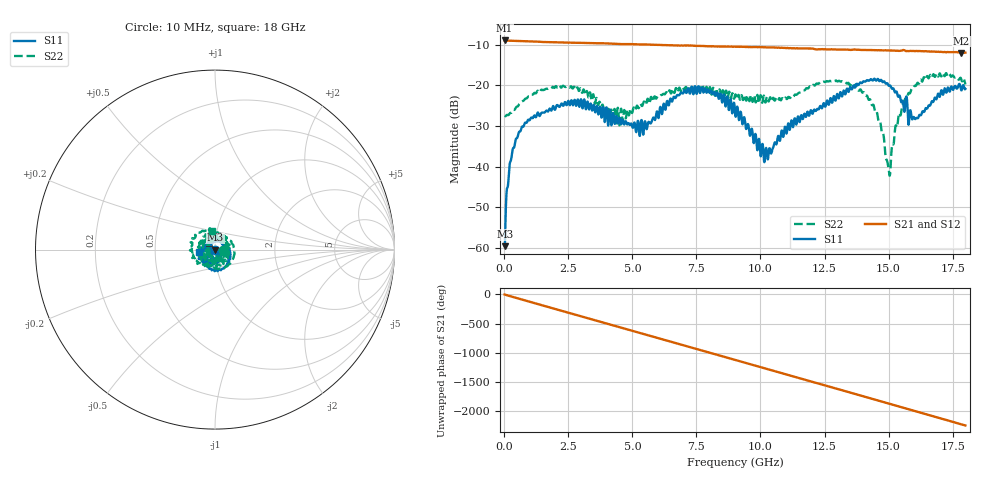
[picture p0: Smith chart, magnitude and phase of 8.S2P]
!Agilent Technologies,E5071C,MY46316741,A.11.02
!Date: Fri May 06 15:19:51 2022
!Data & Calibration Information:
!Freq	S11:SOLT2(ON)	S21:SOLT2(ON)	S12:SOLT2(ON)	S22:SOLT2(ON)
!PortZ  Port1:50+j0  Port2:50+j0
!Above PortZ is port z conversion or system Z0 setting when saving the data.
!When reading, reference impedance value at option line is always used.
# Hz S dB R 50
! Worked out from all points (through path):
!   1800 points, 10 MHz to 18 GHz, reference 50 ohm
!   highest |S21| = -8.93 dB at 10 MHz (marker M1); lowest = -12.0 dB at 17.84 GHz (marker M2)
!   group delay of S21, straight-line fit = 346 ps
!   lowest |S11| = -59.6 dB at 20 MHz (marker M3), VSWR 1.00, Z = 50.1 - j0.0653 ohm
!   |S11| at or under -10 dB: start of sweep to end of sweep
!   |S22| runs from -42.2 to -17.0 dB; largest |S21 - S12| = 0.021
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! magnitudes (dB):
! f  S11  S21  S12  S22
! 10 MHz  -59.1  -8.9  -8.9  -27.5
! 20 MHz  -59.6  -8.9  -8.9  -27.5
! 150 MHz  -44.1  -9.0  -9.0  -27.3
! 260 MHz  -38.3  -9.0  -9.0  -26.7
! 640 MHz  -31.1  -9.1  -9.1  -24.4
! 3.01 GHz  -23.8  -9.5  -9.5  -21.4
! 4.43 GHz  -29.4  -9.8  -9.8  -25.5
! 5.35 GHz  -28.5  -9.9  -9.9  -24.9
! 6.01 GHz  -27.9  -10.0  -10.0  -22.6
! 7.51 GHz  -22.1  -10.3  -10.3  -20.5
! 9.01 GHz  -26.7  -10.5  -10.5  -22.3
! 10.22 GHz  -35.4  -10.6  -10.7  -23.6
! 12.01 GHz  -26.7  -10.9  -11.0  -20.2
! 13.13 GHz  -21.7  -11.2  -11.2  -19.1
! 14.1 GHz  -19.0  -11.3  -11.3  -22.5
! 14.61 GHz  -18.6  -11.3  -11.4  -28.7
! 15.01 GHz  -20.1  -11.4  -11.4  -40.8
! 15.34 GHz  -22.1  -11.5  -11.5  -30.1
! 15.96 GHz  -27.9  -11.5  -11.6  -20.8
! 16.81 GHz  -23.0  -11.7  -11.8  -17.9
! 17.84 GHz  -21.2  -12.0  -12.1  -18.5
! 18 GHz  -20.8  -11.9  -12.1  -19.8
